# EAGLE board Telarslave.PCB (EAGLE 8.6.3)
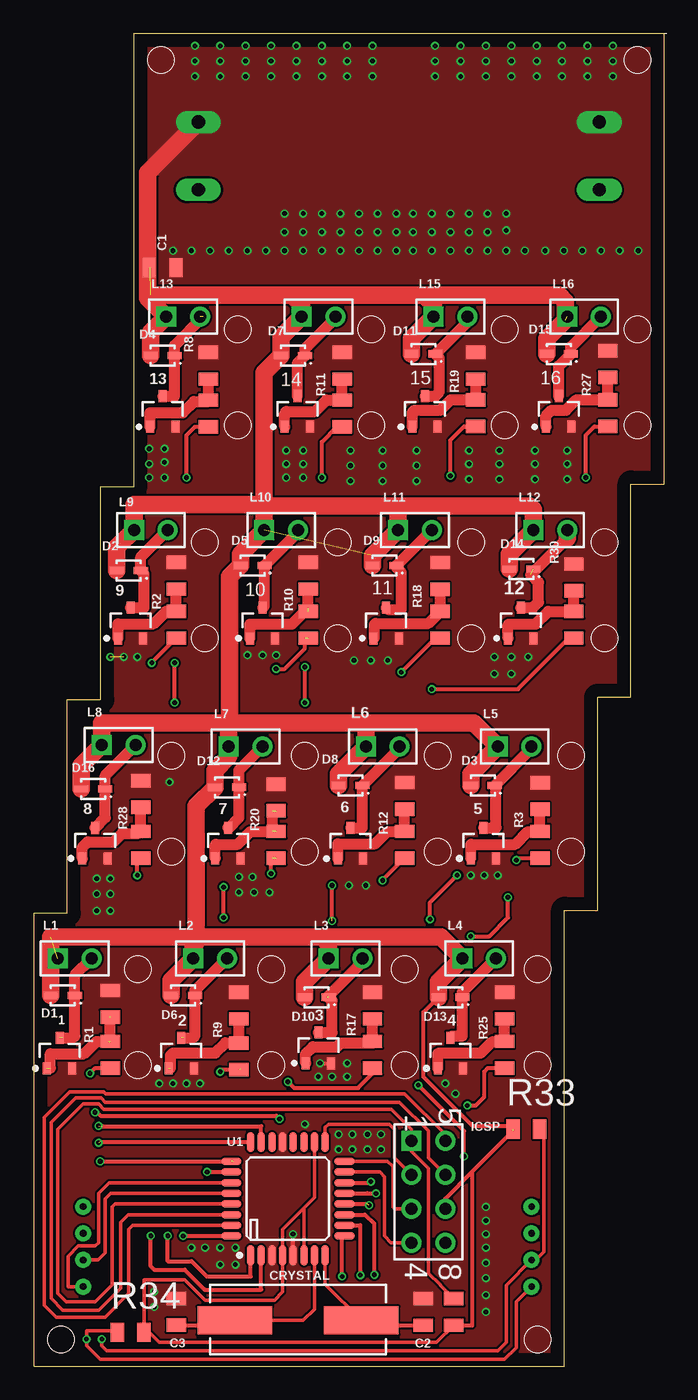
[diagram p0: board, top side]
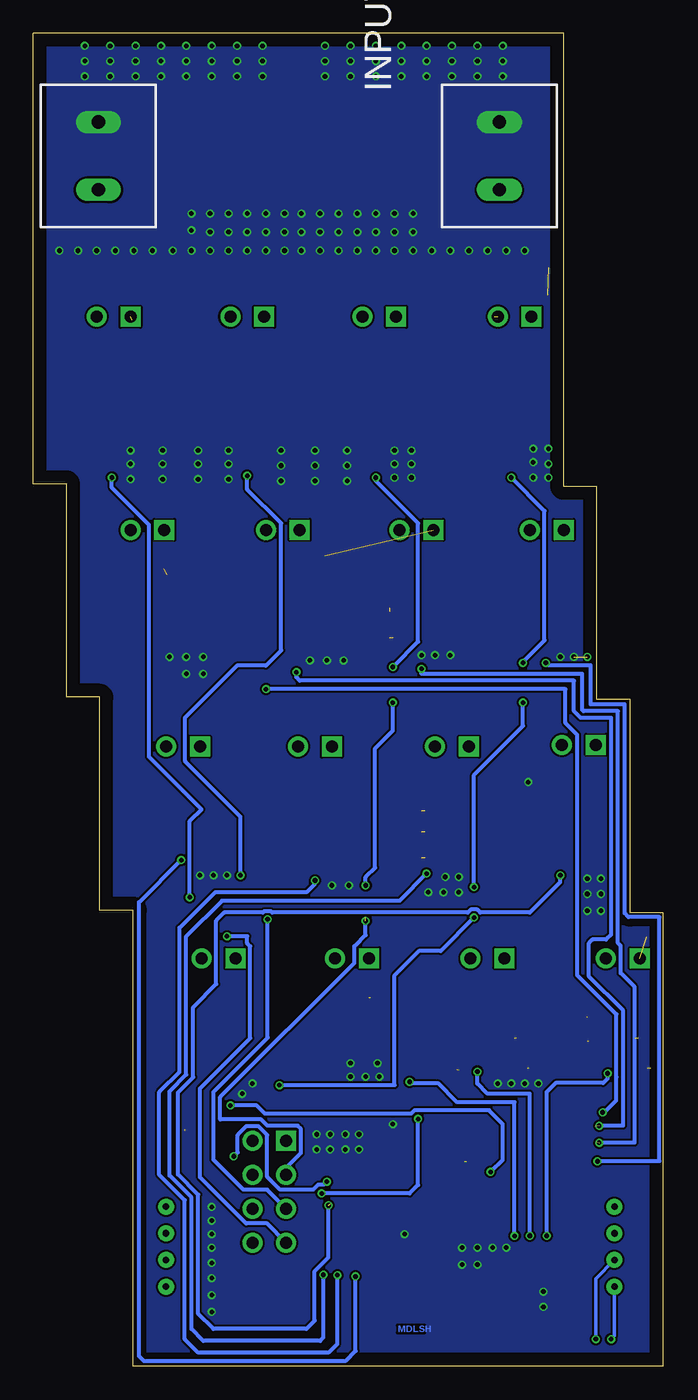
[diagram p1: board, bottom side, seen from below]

Size 47.3 x 100 mm. Coordinates in mm from the lower left corner, seen from the top.
Outline: 7.5,100 47.3,100 47.3,66.2 44.8,66.2 44.8,50.2 42.3,50.2 42.3,34.2 39.8,34.2 39.8,0 0,0 0,34 2.5,34 2.5,50 5,50 5,66 7.5,66 7.5,100
Copper layers (1*16): Top 0.035mm / dielectric 1.5mm / Bottom 0.035mm
Design rules "Telarslave": minimum track width 6mil, minimum drill 0.35mm, track to track 6mil, track to pad 6mil, pad to pad 6mil, via to via 6mil, smd to smd 6mil, copper to edge 40mil, drill to drill 6mil, minimum pad ring 0mil, minimum via ring 0mil, stop-mask expansion 4mil, vias tented up to drill 0mil, thermal gap 10mil

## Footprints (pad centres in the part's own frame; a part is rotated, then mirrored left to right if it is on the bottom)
SOT-23_1PRIMARY = smd 0.9 x 0.6: 1 -1.15,0.95; 2 -1.15,-0.95; 3 1.15,0
RESC0805-I_1PRIMARY = smd 1 x 1.45: 1 -1,0; 2 1,0
CAPC0805-I_1PRIMARY = smd 1 x 1.45: 1 -1,0; 2 1,0
HC49/US_1PRIMARY = smd 5.6 x 2.1: 1 -4.75,0; 2 4.75,0
SODFL250X110-2N_1PRIMARY = smd 1.06 x 0.54: 1 -0.9,0; 2 0.9,0
GROVE90_1PRIMARY = drill 0.5 pad 1.2: 1 -3,0; 2 -1,0; 3 1,0; 4 3,0
HDR2X4_CEN_1PRIMARY = drill 0.9 pad 1.5 square: 1 0,0 | drill 0.9 pad 1.5: 2 2.54,0; 3 5.08,0; 4 7.62,0; 5 0,2.54; 6 2.54,2.54; 7 5.08,2.54; 8 7.62,2.54
2PIN_1PRIMARY = drill 1 pad 1.702 long: 1 0,0; 2 5.08,0
HDR1X2_1PRIMARY = drill 0.9 pad 1.5 square: 1 0,0 | drill 0.9 pad 1.5: 2 2.54,0
TQFP-32_1PRIMARY = smd 1.5 x 0.55: 1 -4.25,2.8; 2 -4.25,2; 3 -4.25,1.2; 4 -4.25,0.4; 5 -4.25,-0.4; 6 -4.25,-1.2; 7 -4.25,-2; 8 -4.25,-2.8; 17 4.25,-2.8; 18 4.25,-2; 19 4.25,-1.2; 20 4.25,-0.4; 21 4.25,0.4; 22 4.25,1.2; 23 4.25,2; 24 4.25,2.8 | smd 0.55 x 1.5: 9 -2.8,-4.25; 10 -2,-4.25; 11 -1.2,-4.25; 12 -0.4,-4.25; 13 0.4,-4.25; 14 1.2,-4.25; 15 2,-4.25; 16 2.8,-4.25; 25 2.8,4.25; 26 2,4.25; 27 1.2,4.25; 28 0.4,4.25; 29 -0.4,4.25; 30 -1.2,4.25; 31 -2,4.25; 32 -2.8,4.25

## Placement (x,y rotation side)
1  Mosfet_N  [SOT-23_1PRIMARY]  1.91,23.5 90 top
2  Mosfet_N  [SOT-23_1PRIMARY]  11.05,23.5 90 top
3  Mosfet_N  [SOT-23_1PRIMARY]  21.34,23.88 90 top
4  Mosfet_N  [SOT-23_1PRIMARY]  31.24,23.5 90 top
5  Mosfet_N  [SOT-23_1PRIMARY]  33.72,39.25 90 top
6  Mosfet_N  [SOT-23_1PRIMARY]  23.75,39.24 90 top
7  Mosfet_N  [SOT-23_1PRIMARY]  14.54,39.25 90 top
8  Mosfet_N  [SOT-23_1PRIMARY]  4.57,39.24 90 top
9  Mosfet_N  [SOT-23_1PRIMARY]  7.24,55.75 90 top
10  Mosfet_N  [SOT-23_1PRIMARY]  17.15,55.75 90 top
11  Mosfet_N  [SOT-23_1PRIMARY]  26.42,55.75 90 top
12  Mosfet_N  [SOT-23_1PRIMARY]  36.52,55.76 90 top
13  Mosfet_N  [SOT-23_1PRIMARY]  9.65,71.63 90 top
14  Mosfet_N  [SOT-23_1PRIMARY]  19.75,71.63 90 top
15  Mosfet_N  [SOT-23_1PRIMARY]  29.34,71.63 90 top
16  Mosfet_N  [SOT-23_1PRIMARY]  39.37,71.63 90 top
C1  100nf  [RESC0805-I_1PRIMARY]  9.65,82.42 0 top
C2  22pf  [CAPC0805-I_1PRIMARY]  29.21,4.06 270 top
C3  22pf  [CAPC0805-I_1PRIMARY]  10.67,4.08 270 top
CRYSTAL  Value  [HC49/US_1PRIMARY]  19.81,3.43 180 top
D1  Diode  [SODFL250X110-2N_1PRIMARY]  2.16,27.81 180 top
D2  Diode  [SODFL250X110-2N_1PRIMARY]  7.11,59.69 180 top
D3  Diode  [SODFL250X110-2N_1PRIMARY]  33.67,43.56 180 top
D4  Diode  [SODFL250X110-2N_1PRIMARY]  9.64,75.82 180 top
D5  Diode  [SODFL250X110-2N_1PRIMARY]  16.38,60.07 180 top
D6  Diode  [SODFL250X110-2N_1PRIMARY]  11.18,27.81 180 top
D7  Diode  [SODFL250X110-2N_1PRIMARY]  19.43,75.82 180 top
D8  Diode  [SODFL250X110-2N_1PRIMARY]  23.75,43.56 180 top
D9  Diode  [SODFL250X110-2N_1PRIMARY]  26.29,60.07 180 top
D10  Diode  [SODFL250X110-2N_1PRIMARY]  21.21,27.69 180 top
D11  Diode  [SODFL250X110-2N_1PRIMARY]  29.21,75.95 180 top
D12  Diode  [SODFL250X110-2N_1PRIMARY]  14.48,43.43 180 top
D13  Diode  [SODFL250X110-2N_1PRIMARY]  31.24,27.69 180 top
D14  Diode  [SODFL250X110-2N_1PRIMARY]  36.58,59.82 180 top
D15  Diode  [SODFL250X110-2N_1PRIMARY]  39.37,75.95 180 top
D16  Diode  [SODFL250X110-2N_1PRIMARY]  4.43,43.31 180 top
I2C  [GROVE90_1PRIMARY]  3.68,8.97 90 bottom
I2C.2  [GROVE90_1PRIMARY]  37.34,8.97 90 bottom
ICSP  [HDR2X4_CEN_1PRIMARY]  28.32,16.89 270 top
INPUT  [2PIN_1PRIMARY]  12.32,88.27 90 bottom
L1  [HDR1X2_1PRIMARY]  1.78,30.61 0 top
L2  [HDR1X2_1PRIMARY]  11.94,30.61 0 top
L3  [HDR1X2_1PRIMARY]  22.1,30.61 0 top
L4  [HDR1X2_1PRIMARY]  32.13,30.61 0 top
L5  [HDR1X2_1PRIMARY]  34.8,46.48 0 top
L6  [HDR1X2_1PRIMARY]  24.89,46.48 0 top
L7  [HDR1X2_1PRIMARY]  14.61,46.48 0 top
L8  [HDR1X2_1PRIMARY]  5.08,46.61 0 top
L9  [HDR1X2_1PRIMARY]  7.49,62.74 0 top
L10  [HDR1X2_1PRIMARY]  17.27,62.74 0 top
L11  [HDR1X2_1PRIMARY]  27.3,62.74 0 top
L12  [HDR1X2_1PRIMARY]  37.47,62.74 0 top
L13  [HDR1X2_1PRIMARY]  9.91,78.74 0 top
L14  [HDR1X2_1PRIMARY]  20.07,78.74 0 top
L15  [HDR1X2_1PRIMARY]  29.97,78.74 0 top
L16  [HDR1X2_1PRIMARY]  40.01,78.74 0 top
OUTPUT  [2PIN_1PRIMARY]  42.42,93.34 270 bottom
R1  1k  [RESC0805-I_1PRIMARY]  5.71,23.37 270 top
R2  1k  [RESC0805-I_1PRIMARY]  10.67,55.63 270 top
R3  1k  [RESC0805-I_1PRIMARY]  37.97,39.12 270 top
R4  1k  [RESC0805-I_1PRIMARY]  13.08,71.49 270 top
R5  220k  [RESC0805-I_1PRIMARY]  5.71,27.19 90 top
R6  220k  [RESC0805-I_1PRIMARY]  10.67,59.31 90 top
R7  220k  [RESC0805-I_1PRIMARY]  37.97,42.78 90 top
R8  220k  [RESC0805-I_1PRIMARY]  13.08,75.06 90 top
R9  1k  [RESC0805-I_1PRIMARY]  15.37,23.24 270 top
R10  1k  [RESC0805-I_1PRIMARY]  20.57,55.63 270 top
R11  1k  [RESC0805-I_1PRIMARY]  23.11,71.49 270 top
R12  1k  [RESC0805-I_1PRIMARY]  27.81,39.12 270 top
R13  220k  [RESC0805-I_1PRIMARY]  15.37,27.05 90 top
R14  220k  [RESC0805-I_1PRIMARY]  20.57,59.31 90 top
R15  220k  [RESC0805-I_1PRIMARY]  23.11,75.06 90 top
R16  220k  [RESC0805-I_1PRIMARY]  27.81,42.8 90 top
R17  1k  [RESC0805-I_1PRIMARY]  25.4,23.37 270 top
R18  1k  [RESC0805-I_1PRIMARY]  30.48,55.63 270 top
R19  1k  [RESC0805-I_1PRIMARY]  33.15,71.5 270 top
R20  1k  [RESC0805-I_1PRIMARY]  18.16,39.12 270 top
R21  220k  [RESC0805-I_1PRIMARY]  25.4,27.05 90 top
R22  220k  [RESC0805-I_1PRIMARY]  30.48,59.29 90 top
R23  220k  [RESC0805-I_1PRIMARY]  33.15,75.06 90 top
R24  220k  [RESC0805-I_1PRIMARY]  18.16,42.67 90 top
R25  1k  [RESC0805-I_1PRIMARY]  35.31,23.37 270 top
R26  1k  [RESC0805-I_1PRIMARY]  40.51,55.63 270 top
R27  1k  [RESC0805-I_1PRIMARY]  43.05,71.5 270 top
R28  1k  [RESC0805-I_1PRIMARY]  8,39.12 270 top
R29  220k  [RESC0805-I_1PRIMARY]  35.31,27.05 90 top
R30  220k  [RESC0805-I_1PRIMARY]  40.51,59.18 90 top
R31  220k  [RESC0805-I_1PRIMARY]  43.05,75.18 90 top
R32  220k  [RESC0805-I_1PRIMARY]  8,42.93 90 top
R33  4.7K  [RESC0805-I_1PRIMARY]  36.94,17.78 180 top
R34  4.7k  [RESC0805-I_1PRIMARY]  7.24,2.54 0 top
R35  10K  [RESC0805-I_1PRIMARY]  31.5,4.06 90 top
U1  ATmega328P-AU  [TQFP-32_1PRIMARY]  19.05,12.57 90 top

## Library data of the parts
1-16 C1-C3 CRYSTAL D1-D16 I2C I2C.2 ICSP INPUT L1-L16 OUTPUT R1-R35 U1 = Telarslave

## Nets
5V: C1.1 D1.2 D2.2 D3.2 D4.2 D5.2 D6.2 D7.2 D8.2 D9.2 D10.2 D11.2 D12.2 D13.2 D14.2 D15.2 D16.2 ICSP.7 INPUT.2 L1.1 L2.1 L3.1 L4.1 L5.1 L6.1 L7.1 L8.1 L9.1 L10.1 L11.1 L12.1 L13.1 L14.1 L15.1 L16.1 OUTPUT.1 R33.2 R34.2 R35.1 U1.4 U1.6 U1.18
B1: R1.2 U1.2
B2: R9.2 U1.1
B3: R17.2 U1.32
B4: R25.2 U1.26
B5: R3.2 U1.9
B6: R12.2 U1.10
B7: R20.2 U1.11
B8: R28.2 U1.12
B9: R2.2 U1.25
B10: R10.2 U1.24
B11: R18.2 U1.23
B12: R26.2 U1.13
B13: R4.2 U1.14
B14: ICSP.2 R11.2 U1.17
B15: ICSP.3 R19.2 U1.16
B16: ICSP.4 R27.2 U1.15
GND: 1.2 2.2 3.2 4.2 5.2 6.2 7.2 8.2 9.2 10.2 11.2 12.2 13.2 14.2 15.2 16.2 C1.2 C2.1 C3.1 R5.2 R6.2 R7.2 R8.2 R13.2 R14.2 R15.2 R16.2 R21.2 R22.2 R23.2 R24.2 R29.2 R30.2 R31.2 R32.2 U1.3 U1.5 U1.21
NET1_1: 1.1 R1.1 R5.1
NET1_3: 1.3 D1.1 L1.2
NET2_1: 2.1 R9.1 R13.1
NET2_3: 2.3 D6.1 L2.2
NET3_1: 3.1 R17.1 R21.1
NET3_3: 3.3 D10.1 L3.2
NET4_1: 4.1 R25.1 R29.1
NET4_3: 4.3 D13.1 L4.2
NET5_1: 5.1 R3.1 R7.1
NET5_3: 5.3 D3.1 L5.2
NET6_1: 6.1 R12.1 R16.1
NET6_3: 6.3 D8.1 L6.2
NET7_1: 7.1 R20.1 R24.1
NET7_3: 7.3 D12.1 L7.2
NET8_1: 8.1 R28.1 R32.1
NET8_3: 8.3 D16.1 L8.2
NET9_1: 9.1 R2.1 R6.1
NET9_3: 9.3 D2.1 L9.2
NET10_1: 10.1 R10.1 R14.1
NET10_3: 10.3 D5.1 L10.2
NET11_1: 11.1 R18.1 R22.1
NET11_3: 11.3 D9.1 L11.2
NET12_1: 12.1 R26.1 R30.1
NET12_3: 12.3 D14.1 L12.2
NET13_1: 13.1 R4.1 R8.1
NET13_3: 13.3 D4.1 L13.2
NET14_1: 14.1 R11.1 R15.1
NET14_3: 14.3 D7.1 L14.2
NET15_1: 15.1 R19.1 R23.1
NET15_3: 15.3 D11.1 L15.2
NET16_1: 16.1 R27.1 R31.1
NET16_3: 16.3 D15.1 L16.2
NETC2_2: C2.2 CRYSTAL.1 U1.8
NETC3_2: C3.2 CRYSTAL.2 U1.7
RESET: ICSP.1 R35.2 U1.29
RXD: ICSP.6 U1.30
SCL: R33.1 U1.28
SDA: R34.1 U1.27
TXD: ICSP.5 U1.31

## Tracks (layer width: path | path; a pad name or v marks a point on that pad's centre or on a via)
5V  (via drill 0.35 pad 0.6)  (5 unrouted)
  Top 0.254: R35.1 30.21,1.78 9.4,1.78 8.64,2.54 R34.2 8.26,2.56 8.26,6.48 11.3,6.48 12.83,4.95 18.03,4.95 18.65,5.57 U1.4 18.65,10.27 20.25,11.87 | 20.25,11.87 21.05,12.67 U1.18 | U1.6 20.25,11.87
  Top 0.305: 32.89,14.61 30.86,12.57 ICSP.7 | 32.89,14.61 35.94,17.65 35.56,18.03 32.89,18.03 29.21,21.72 29.21,26.55 D13.2 | 32.89,14.61 32.89,3.06 R35.1
  Top 1.321: 8.51,80.14 8.51,89.53 INPUT.2 | D1.2 1.26,32.22 12.16,32.22 | 17.27,64.52 17.27,74.56 D7.2 18.53,77.21 L14.1 20.07,79.63 19.34,80.35 | D11.2 28.31,77.08 L15.1 29.97,79.63 29.25,80.35 | D15.2 38.47,77.08 39.88,78.49 39.88,79.88 39.41,80.35 29.25,80.35 | 19.34,80.35 29.25,80.35 | 19.34,80.35 8.73,80.35 8.51,80.14 | D4.2 8.74,77.57 L13.1 8.51,80.14 | 14.61,48.26 5.08,48.26 L8.1 3.53,45.06 D16.2 | 14.61,48.26 24.51,48.26 | 24.51,48.26 33.02,48.26 L5.1 32.77,44.45 D3.2 | 24.51,48.26 24.89,47.88 L6.1 22.85,44.44 D8.2 | D14.2 35.68,60.95 L12.1 37.47,64.26 37.21,64.52 17.27,64.52 | D9.2 25.39,60.82 L11.1 27.3,64.13 | 14.61,48.26 14.66,48.32 14.66,59.25 D5.2 15.48,60.95 L10.1 17.27,64.52 | 17.27,64.52 17.15,64.64 7.49,64.64 L9.1 6.21,61.46 D2.2 | 12.16,32.22 21.59,32.22 | 21.59,32.22 30.52,32.22 L4.1 30.34,28.82 D13.2 | 12.16,32.22 12.16,42.02 D12.2 13.58,44.71 14.61,45.74 L7.1 14.61,48.26 | 12.16,32.22 12.16,31.81 11.94,31.59 L2.1 10.28,28.95 D6.2 | D10.2 20.31,28.82 L3.1 22.1,31.71 21.59,32.22
  other vias: 30.1,99.06 30.1,97.92 30.1,96.77 32,99.06 32,97.92 32,96.77 35.81,96.77 35.81,97.92 35.81,99.06 33.91,96.77 33.91,97.92 33.91,99.06 41.53,99.06 41.53,97.92 41.53,96.77 43.43,99.06 43.43,97.92 43.43,96.77 39.62,96.77 39.62,97.92 39.62,99.06 37.72,96.77 37.72,97.92 37.72,99.06 19.69,99.06 19.69,97.92 19.69,96.77 21.59,99.06 21.59,97.92 21.59,96.77 25.4,96.77 25.4,97.92 25.4,99.06 23.5,96.77 23.5,97.92 23.5,99.06 15.88,99.06 15.88,97.92 15.88,96.77 17.78,99.06 17.78,97.92 17.78,96.77 13.97,96.77 13.97,97.92 13.97,99.06 12.07,96.77 12.07,97.92 12.07,99.06
  pour Top (no thermals): 7.5,89.41 7.5,100 47.3,100 47.3,89.41
  pour Bottom (no thermals): 7.5,89.41 7.5,100 47.3,100 47.3,89.41
B1  (via drill 0.35 pad 0.6)
  Top 0.305: v8.76,9.78 8.76,7.49 9.02,7.24 11.3,7.24 12.8,5.75 17.05,5.75 U1.2 | v4.19,21.97 4.59,22.37 R1.2
  Bottom 0.305: v4.19,21.97 4.19,21.59 4.54,21.25 8.09,21.25 8.76,20.57 v8.76,9.78
B2  (via drill 0.35 pad 0.6)  (1 unrouted)
  Top 0.305: 15.49,22.26 14,22.26 13.97,22.23 v13.97,22.1 | v10.03,9.78 10.03,7.87 11.81,7.87 12.95,6.74 16.25,6.74 U1.1
  Bottom 0.305: v13.97,22.1 13.97,21.21 13.21,20.45 10.03,20.45 v10.03,9.78
B3  (via drill 0.35 pad 0.6)
  Top 0.305: R17.2 25.4,21.97 24.31,20.88 19.51,20.88 v19.05,21.34 | v11.18,9.77 U1.32
  Bottom 0.305: v11.18,9.77 11.18,19.81 15.49,19.81 16.89,21.21 18.92,21.21 v19.05,21.34
B4  (via drill 0.35 pad 0.6)
  Top 0.305: v32.51,19.56 33.15,19.56 33.78,20.19 33.78,22.1 34.05,22.37 R25.2 | v12.99,14.57 U1.26
  Bottom 0.305: v32.51,19.56 30.53,19.56 29.91,18.94 18.94,18.94 18.69,19.2 13.1,19.2 12.07,18.16 12.07,15.49 v12.99,14.57
B5  (via drill 0.35 pad 0.6)
  Top 0.305: R3.2 36.34,38.12 v36.2,37.97 | v23.11,6.73 23.11,9.59 U1.9
  Bottom 0.305: v36.2,37.97 39.37,34.8 39.37,0.76 38.99,0.38 23.88,0.38 23.11,1.14 v23.11,6.73
B6  (via drill 0.35 pad 0.6)
  Top 0.305: 26.16,36.47 R12.2 | v24.48,6.83 24.48,10.57 U1.10
  Top 0.406: v26.16,36.45 26.16,36.47
  Bottom 0.305: v26.16,36.45 26.16,36.2 26.8,35.56 33.66,35.56 36.32,32.89 36.32,22.1 37.85,20.57 37.85,14.35 35.94,12.45 35.94,2.03 34.93,1.02 25.15,1.02 24.48,1.68 v24.48,6.83
B7  (via drill 0.35 pad 0.6)  (1 unrouted)
  Top 0.305: v17.78,36.96 17.78,37.96 17.76,37.97 17.91,38.12 | v25.53,6.86 25.53,10.67 24.82,11.37 U1.11
  Bottom 0.305: v17.78,36.96 19.81,34.93 33.15,34.93 35.81,32.26 35.81,21.89 37.08,20.62 37.08,14.31 35.43,12.66 35.43,2.79 34.54,1.91 25.78,1.91 25.53,2.16 v25.53,6.86
B8  (via drill 0.35 pad 0.6)  (1 unrouted)
  Top 0.305: R28.2 7.75,37.86 v7.75,36.83 | U1.12 25,12.17
  Bottom 0.305: v7.75,36.83 7.75,36.32 10.03,34.04 13.75,34.04 13.97,34.26 14.48,34.26 14.7,34.04 29.37,34.04 29.47,34.13 29.97,34.13 30.07,34.04 32.97,34.04 33.57,33.44 33.57,28.66 35.31,26.92 35.31,21.68 36.45,20.53 36.45,14.39 34.93,12.87 34.93,3.94 33.78,2.79 26.8,2.79 26.18,3.41 26.18,7.13 25.15,8.17 v25.15,12.07
B9  (via drill 0.35 pad 0.6)  (1 unrouted)
  Top 0.305: R2.2 8.83,52.78 v8.83,52.77 | v4.96,15.37 14.93,15.37
  Bottom 0.305: v8.83,52.77 8.64,52.58 5.46,52.58 5.46,49.66 2.92,49.66 2.92,33.99 2.63,33.7 0.3,33.7 0.3,15.37 v4.96,15.37
B10  (via drill 0.35 pad 0.6)  (2 unrouted)
  Top 0.305: v18.16,52.32 18.8,52.32 20.32,53.85 20.32,54.63 | 5.01,16.82 U1.24
  Bottom 0.305: v18.16,52.32 18.16,51.94 6.1,51.94 6.1,49.23 6.01,49.15 3.43,49.15 3.43,31.75 3.21,31.54 3.21,29.5 2.16,28.45 2.16,16.76 v4.83,16.76
B11  (via drill 0.35 pad 0.6)  (1 unrouted)
  Top 0.305: R18.2 30.12,54.63 v27.56,52.07 | U1.23 17.05,18 5.11,18
  Bottom 0.305: v4.83,18.03 3.03,18.03 3.03,26.68 5.59,29.24 5.59,31.75 5.33,32 4.32,32 3.94,32.38 3.94,48.64 6.22,48.64 6.73,49.15 6.73,51.43 27.3,51.43 27.56,51.69 v27.56,52.07
B12  (via drill 0.35 pad 0.6)
  Top 0.305: v18.41,18.54 18.16,18.8 4.99,18.8 4.74,19.05 v4.57,19.05 | v29.84,50.8 36.32,50.8 40.15,54.63 R26.2 | v25.65,12.95 25.02,12.95 25,12.97 U1.13
  Bottom 0.305: v29.84,50.8 7.37,50.8 7.37,48.26 6.48,47.37 6.48,29.34 3.54,26.4 3.54,21.7 3.56,21.68 3.56,19.94 4.45,19.05 v4.57,19.05 | v18.41,18.54 18.41,13.59 19.05,12.95 v25.65,12.95
B13  (via drill 0.35 pad 0.6)
  Top 0.305: v32.26,15.75 32.26,17.65 v28.83,21.08 | v25.27,13.84 25.2,13.77 U1.14 | v14.22,33.66 v14.22,35.94 | v10.54,49.78 v10.54,52.77 | v11.43,66.68 11.43,69.85 12.07,70.49 R4.2
  Bottom 0.305: v11.43,66.68 8.93,64.17 8.93,54.45 10.54,52.83 v10.54,52.77 | v32.26,15.75 31.97,16.04 31.97,17.35 31.32,18 30.4,18 29.76,17.35 29.76,14.22 28.78,13.25 26.29,13.25 25.93,13.61 25.51,13.61 v25.27,13.84 | v28.83,21.08 20.19,21.08 20.19,29.32 18.36,31.16 16.72,31.16 v14.22,33.66 | v14.22,35.94 14.22,44.36 10.54,48.04 v10.54,49.78
B14  (via drill 0.35 pad 0.6)  (1 unrouted)
  Top 0.254: ICSP.2 27.05,15.62 27.05,17.78 26.68,18.15 22.1,18.15 21.85,17.9 U1.17
  Top 0.305: 22.35,33.66 v22.35,36.07 | v20.32,49.78 v20.32,52.45 | v21.59,66.68 21.59,69.34 22.73,70.49 R11.2
  Bottom 0.305: v20.32,52.45 18.41,54.36 18.41,63.25 21.59,66.42 v21.59,66.68 | ICSP.2 28.32,14.89 27.22,15.99 27.22,17.79 27.46,18.03 29.72,18.03 30.19,18.51 33.27,18.51 33.27,20.19 23.2,30.26 23.2,31.5 22.35,32.36 v22.35,33.4 | v22.35,36.07 22.35,36.7 21.66,37.4 21.66,46.36 20.32,47.7 v20.32,49.78
B15  (via drill 0.35 pad 0.6)
  Top 0.254: ICSP.3 27.05,11.81 26.92,11.94 26.92,14.99 26.54,15.37 U1.16
  Top 0.305: v29.72,33.53 29.72,34.8 v31.75,36.83 | v31.24,66.8 31.24,69.47 32.27,70.5 R19.2
  Bottom 0.305: v31.24,66.8 31.24,65.79 28.7,63.25 28.7,53.7 29.84,52.56 32.02,52.56 35.9,48.68 35.9,45.38 31.75,41.22 v31.75,36.83 | ICSP.3 29.76,13.25 31.53,13.25 33.78,15.49 33.78,20.57 29.72,24.64 v29.72,33.53
B16  (via drill 0.35 pad 0.6)
  Top 0.254: U1.15 25.94,14.57 26.29,14.22 26.29,9.78 26.8,9.27 ICSP.4
  Top 0.305: v35.56,35.18 35.56,33.66 34.16,32.26 v32.77,32.26 | v41.4,66.68 41.4,69.85 42.05,70.5 R27.2
  Bottom 0.305: v35.56,35.18 35.56,40.89 34.67,41.78 38.61,45.72 38.61,63.12 41.4,65.91 v41.4,66.68 | ICSP.4 29.76,10.7 31.32,10.7 34.8,14.18 34.8,20.83 31.02,24.6 31.02,31.5 31.24,31.72 31.24,32.26 v32.77,32.26
GND  (via drill 0.35 pad 0.6)  (1 unrouted)
  Top 0.305: v19.43,9.91 19.45,9.89 U1.5 | v21.46,22.73 v21.47,22.73 3.2
  other vias: 9.02,4.45 9.02,5.59 33.91,4.06 33.91,5.33 33.91,6.6 33.91,7.75 33.91,8.89 33.91,10.92 33.91,11.94 13.97,7.62 15.11,7.62 11.81,8.89 12.83,8.89 13.97,8.89 15.11,8.89 22.86,16.26 23.88,16.26 25.02,16.26 26.04,16.26 26.04,17.4 25.02,17.4 23.88,17.4 22.86,17.4 31.62,20.45 30.86,21.21 12.45,21.21 11.43,21.21 10.41,21.21 9.4,21.21 23.5,22.73 23.5,21.72 22.35,21.72 21.34,21.72 34.8,36.83 33.78,36.83 32.77,36.83 24.89,36.07 23.62,36.07 5.71,34.16 4.7,34.16 4.7,35.43 5.71,35.43 5.71,36.58 4.7,36.58 35.81,51.94 34.54,51.94 37.08,53.21 35.81,53.21 34.54,53.21 26.54,52.96 25.27,52.96 24,52.96 18.16,53.34 17.15,53.34 6.73,53.21 5.71,53.21 17.65,35.56 16.51,35.56 15.37,35.56 16.38,36.7 15.37,36.7 40.01,66.55 40.01,67.69 40.01,68.71 37.59,66.55 37.59,67.69 37.59,68.71 34.93,66.55 34.93,67.69 34.93,68.71 32.64,66.55 32.64,67.69 32.64,68.71 28.7,66.42 26.16,66.42 23.75,66.42 23.75,67.56 26.16,67.56 28.7,67.56 28.7,68.71 26.16,68.71 23.75,68.71 20.19,66.68 9.78,66.68 8.64,66.68 18.92,66.68 20.19,67.69 18.92,67.69 20.19,68.71 18.92,68.71 9.78,67.82 9.78,68.83 8.64,68.83 8.64,67.69 10.41,83.69 11.81,83.69 13.21,83.69 14.61,83.69 16,83.69 17.4,83.69 45.34,83.69 43.94,83.69 42.54,83.69 41.15,83.69 39.75,83.69 38.35,83.69 36.83,83.69 18.8,83.69 18.8,85.09 20.19,83.69 20.19,85.09 21.59,83.69 21.59,85.09 22.99,83.69 22.99,85.09 24.38,83.69 24.38,85.09 35.43,83.69 34.04,83.69 32.64,83.69 31.24,83.69 29.84,83.69 28.45,83.69 27.18,83.69 25.78,83.69 25.78,85.09 27.18,85.09 28.45,85.09 29.84,85.09 31.24,85.09 32.64,85.09 34.04,85.09 35.43,85.22 35.43,86.49 34.04,86.49 32.64,86.49 31.24,86.49 29.84,86.49 28.45,86.49 27.18,86.49 25.78,86.49 24.38,86.49 22.99,86.49 21.59,86.49 20.19,86.49 18.8,86.49 33.91,9.91 20.32,18.16 10.16,43.82 7.75,53.21 16,53.34
  pour Top (no thermals): 0.38,0.13 0.38,34.13 2.88,34.13 2.88,50.13 5.38,50.13 5.38,66.13 7.88,66.13 7.88,89.54 47.3,89.54 47.3,66.33 44.58,66.33 44.58,50.33 42.3,50.33 42.3,34.33 39.8,34.33 39.8,0.13
  pour Bottom (no thermals): 0,0.13 39.8,0.13 39.8,34.33 42.3,34.33 42.3,50.33 44.8,50.33 44.8,66.33 47.3,66.33 47.3,89.53 7.5,89.53 7.5,66.13 5.08,66.13 5.08,50.21 5,50.13 2.5,50.13 2.5,34.13 0,34.13
NET1_1  (3 unrouted)
  Top 0.813: R1.1 5.71,26.18 | 5.59,24.37 4.68,24.37 3.75,23.43 1.21,23.43 1.21,22.34
NET1_3  (1 unrouted)
  Top 0.813: L1.2 3.06,29.35 D1.1 3.06,24.78 2.93,24.65 2.16,24.65
NET2_1  (1 unrouted)
  Top 0.305: R9.1 15.37,24.26
  Top 0.813: R13.1 15.37,24.26 14.35,24.26 13.59,23.5 10.41,23.5 10.23,23.31 10.23,22.34
NET2_3  (1 unrouted)
  Top 0.813: L2.2 12.08,28.2 D6.1 12.08,24.79 11.93,24.65 11.18,24.65
NET3_1
  Top 0.813: R21.1 R17.1 25.4,24.24 23.01,24.24 22.74,23.97 20.92,23.97 20.39,23.43 3.1
NET3_3  (1 unrouted)
  Top 0.813: 21.98,27.69 24.64,30.34 L3.2 | D10.1 22.36,27.44 22.36,25.03 3.3
NET4_1
  Top 0.813: 4.1 30.29,23.43 30.35,23.5 33.53,23.5 34.4,24.37 R25.1 R29.1
NET4_3
  Top 0.305: 32.13,27.68 D13.1 | 4.3 31.36,24.77
  Top 0.813: L4.2 32.14,28.08 D13.1 | 32.13,27.68 32.13,24.77 31.36,24.77
NET5_1
  Top 0.813: 5.1 32.77,39.12 32.81,39.16 36.11,39.16 37.07,40.12 R3.1 R7.1
NET5_3
  Top 0.813: L5.2 37.34,46.33 D3.1 34.66,43.47 34.66,40.4 5.3
NET6_1
  Top 0.813: 6.1 22.8,39.18 25.59,39.18 26.53,40.12 R12.1 R16.1
NET6_3
  Top 0.813: L6.2 27.43,46.34 D8.1 24.64,43.55 24.64,40.39 6.3
NET7_1  (2 unrouted)
  Top 0.813: 7.1 13.59,39.11 13.64,39.16 15.28,39.16 16.24,40.12 17.91,40.12 17.91,41.67
NET7_3
  Top 0.813: 7.3 14.62,40.4 15.38,41.16 D12.1 15.38,44.71 L7.2
NET8_1
  Top 0.813: 8.1 3.62,38.93 4.03,39.33 5.96,39.33 6.6,39.97 7.86,39.97 R28.1 R32.1
NET8_3
  Top 0.813: 8.3 5.33,41.16 D16.1 5.33,44.32 L8.2
NET9_1
  Top 0.813: 9.1 6.29,55.69 8.96,55.69 9.89,56.63 R2.1 R6.1
NET9_3
  Top 0.813: L9.2 8.01,60.72 D2.1 8.26,59.45 8.26,56.9 9.3
NET10_1  (1 unrouted)
  Top 0.813: R14.1 20.57,56.88 19.36,55.66 16.2,55.66 10.1
NET10_3
  Top 0.813: 10.3 17.28,57.04 D5.1 19.7,62.48 19.7,62.74 L10.2
NET11_1
  Top 0.305: 11.1 25.53,54.66
  Top 0.813: 25.53,54.66 25.53,55.63 25.64,55.74 29.59,55.74 R18.1 R22.1
NET11_3
  Top 0.813: 11.3 26.55,56.77 27.56,56.77 27.56,59.56 27.19,59.93 D9.1 29.84,62.73 L11.2
NET12_1
  Top 0.813: 12.1 35.57,55.62 35.61,55.67 37.64,55.67 38.59,56.63 R26.1 R30.1
NET12_3  (1 unrouted)
  Top 0.813: 40.01,62.13 37.26,59.38 37.85,58.8 37.85,57.32 37.44,56.91 12.3
  Top 1.321: 40.01,62.13 L12.2
NET13_1
  Top 0.813: R8.1 R4.1 13.08,72.37 11.99,72.37 11.15,71.54 8.7,71.54 13.1
NET13_3  (1 unrouted)
  Top 0.813: 13.3 10.53,72.78 D4.1 10.54,76.58 12.7,78.74
NET14_1
  Top 0.813: 14.1 18.8,71.51 18.92,71.63 21.08,71.63 21.94,72.49 R11.1 R15.1
NET14_3
  Top 0.813: 14.3 19.75,75.24 D7.1 20.33,76.34 22.61,78.61 L14.2
NET15_1
  Top 0.813: 15.1 28.39,71.57 28.54,71.72 30.48,71.72 31.27,72.5 R19.1 R23.1
NET15_3
  Top 0.813: 15.3 30.11,72.78 30.42,73.09 30.42,75.64 D11.1 32.51,78.35 L15.2
NET16_1
  Top 0.813: 16.1 38.42,71.31 38.82,71.72 39.92,71.72 40.71,72.5 R27.1 R31.1
NET16_3
  Top 0.813: L16.2 40.27,76.47 D15.1 39.37,75.05 16.3
NETC2_2
  Top 0.254: U1.8 21.85,6.14 CRYSTAL.1 24.93,3.06
  Top 0.305: 24.93,3.06 C2.2
NETC3_2
  Top 0.254: U1.7 21.05,4.29 20.19,3.43 CRYSTAL.2 14.71,3.08
  Top 0.305: C3.2 14.71,3.08
RESET
  Top 0.254: R35.2 30.48,6.08 30.48,6.1 29.59,6.98 29.59,14.86 28.32,16.13 ICSP.1 28.32,17.78 26.82,19.28 5.24,19.28 4.83,19.68 3.68,19.68 1.78,17.78 1.78,5.46 2.41,4.83 4.57,4.83 5.84,6.1 5.84,11.94 6.08,12.17 U1.29 14.65,12.32
RXD
  Top 0.254: U1.30 7.05,11.37 6.48,10.8 6.48,5.84 4.83,4.19 2.16,4.19 1.27,5.08 1.27,18.29 3.12,20.14 5.02,20.14 5.35,19.81 27.43,19.81 29.59,17.65 29.59,15.62 ICSP.6
SCL  (via drill 0.35 pad 0.6)  (1 unrouted)
  Top 0.254: R33.1 38.27,17.45 38.27,8.57 37.66,7.97 37.34,7.97 35.43,6.06 35.43,1.78 34.8,1.14 5.46,1.14 5.08,1.52 v5.08,2.03 | 3.68,7.97 4.79,7.97 5.33,8.51 5.33,12.57 5.73,12.97 U1.28
  Bottom 0.254: 3.68,7.97 5.08,6.57 v5.08,2.03
SDA  (via drill 0.35 pad 0.6)  (1 unrouted)
  Top 0.254: R34.1 6.12,2.66 3.93,2.66 v3.93,2.04 v3.94,2.03 3.94,1.52 4.95,0.51 35.31,0.51 36.2,1.4 36.2,4.83 37.34,5.97 | 3.68,5.97 2.54,5.97 2.54,8.26 3.3,9.02 4.57,9.02 4.83,9.27 4.83,12.95 5.65,13.77 U1.27
  Bottom 0.254: v3.94,2.03 3.68,2.29 3.68,5.97
TXD
  Top 0.254: ICSP.5 30.86,17.4 27.81,20.45 5.36,20.45 5.21,20.59 2.69,20.59 0.76,18.67 0.76,4.57 1.65,3.68 5.33,3.68 7.11,5.46 7.11,10.29 7.4,10.57 U1.31

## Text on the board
Bottom: MDLSH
